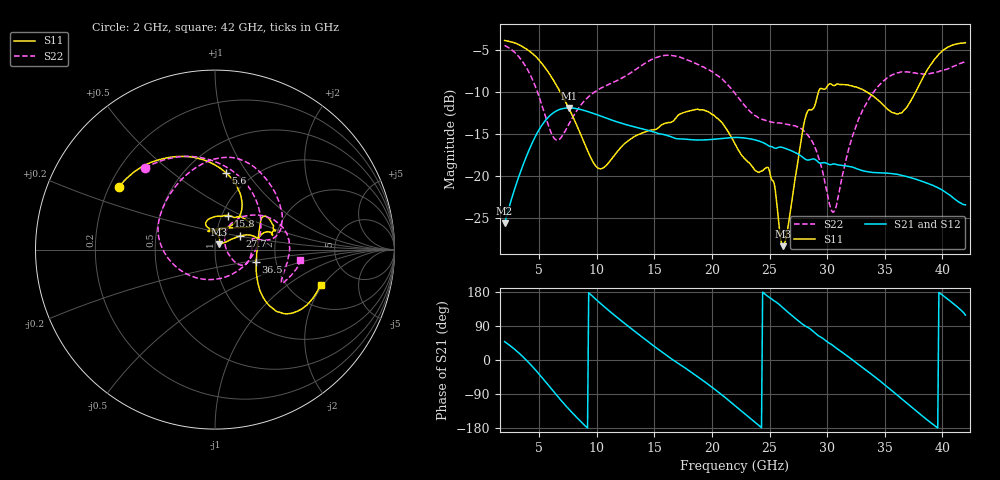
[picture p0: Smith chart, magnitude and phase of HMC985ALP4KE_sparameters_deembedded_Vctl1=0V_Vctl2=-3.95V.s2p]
!s2p File: Measurements: S11, S21, S12, S22
# GHz S dB R 50.0
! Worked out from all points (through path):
!   401 points, 2 GHz to 42 GHz, reference 50 ohm
!   highest |S21| = -11.92 dB at 7.6 GHz (marker M1); lowest = -25.7 dB at 2 GHz (marker M2)
!   lowest |S11| = -28.4 dB at 26.2 GHz (marker M3), VSWR 1.08, Z = 52.3 + j3.16 ohm
!   |S11| at or under -10 dB: 6.822 GHz to 29.25 GHz (22.43 GHz wide, 124 % of centre); 33.42 GHz to 37.69 GHz (4.268 GHz wide, 12 % of centre)
!   |S22| runs from -24.3 to -4.5 dB; largest |S21 - S12| = 0.00021
!   S11 on the Smith chart (normalised r, x): 2 GHz: 0.24, +0.28; 5.6 GHz: 0.76, +0.80; 15.8 GHz: 1.07, +0.42; 27.7 GHz: 1.30, +0.20; 36.5 GHz: 1.57, -0.23; 42 GHz: 2.95, -1.89
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2  -3.88 147.0  -25.68 48.6  -25.69 48.6  -4.47 130.5
3.6  -4.65 120.3  -18.71 8.2  -18.71 8.2  -6.49 85.0
4.6  -5.66 101.5  -15.50 -23.5  -15.50 -23.5  -9.11 47.9
5.6  -7.28 81.8  -13.31 -59.3  -13.32 -59.3  -13.15 -3.6
6.5  -9.21 66.5  -12.27 -92.2  -12.27 -92.2  -15.73 -69.4
7.6  -12.03 54.7  -11.92 -130.3  -11.92 -130.4  -13.79 -136.5
8.7  -15.38 55.0  -12.14 -165.0  -12.14 -165.0  -11.43 -170.7
10.4  -19.16 89.7  -12.91 147.2  -12.92 147.2  -9.53 161.9
15.4  -14.21 75.7  -14.98 27.0  -14.98 27.0  -5.80 86.4
15.8  -13.82 68.7  -15.08 18.1  -15.08 18.1  -5.68 81.4
19.3  -12.17 33.5  -15.72 -55.8  -15.72 -55.9  -7.06 35.7
22  -16.19 51.2  -15.44 -120.5  -15.44 -120.5  -10.19 10.3
24.9  -19.04 104.6  -16.41 166.9  -16.42 166.9  -13.50 13.1
26.2  -28.38 52.3  -16.65 136.5  -16.66 136.5  -13.79 -3.3
27.7  -16.12 28.6  -17.60 98.4  -17.61 98.4  -14.35 -24.2
28.7  -12.11 12.6  -18.00 77.9  -18.00 77.9  -15.90 -31.8
30.6  -9.26 19.6  -18.59 35.9  -18.58 35.9  -24.25 21.6
32.8  -9.58 34.0  -19.27 -14.0  -19.27 -14.0  -13.03 52.0
35.4  -12.22 11.7  -19.71 -75.3  -19.70 -75.4  -8.18 20.3
36.5  -12.47 -16.7  -19.95 -103.3  -19.95 -103.3  -7.62 6.4
39.5  -5.86 -43.7  -21.34 -177.2  -21.36 -177.2  -7.63 -26.0
42  -4.15 -18.5  -23.45 118.4  -23.45 118.3  -6.39 -6.7
